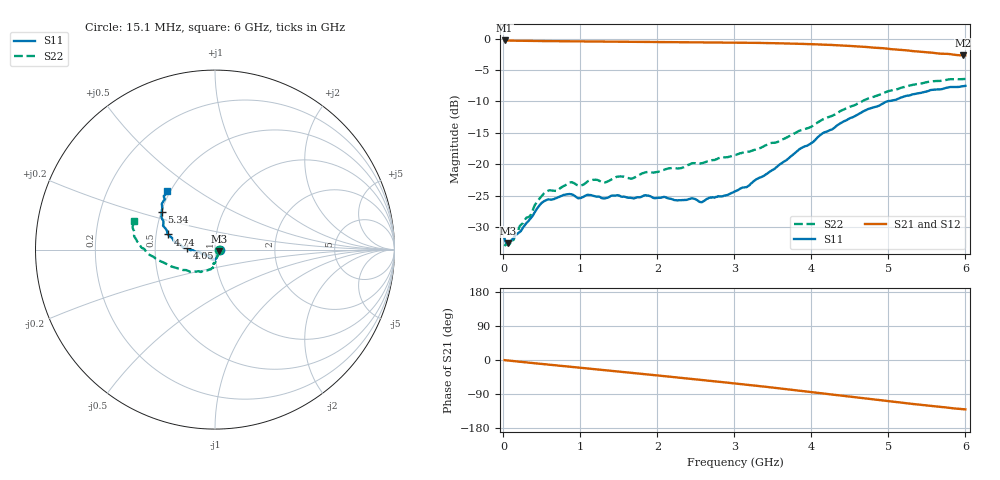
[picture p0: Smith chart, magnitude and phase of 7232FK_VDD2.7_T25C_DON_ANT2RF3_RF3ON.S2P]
!Agilent Technologies,E5071C,MY46417908,A.11.23
!Date: Fri Mar 03 11:30:21 2017
!Data & Calibration Information:
!Freq	S11:SOLT2(ON)	S21:SOLT2(ON)	S12:SOLT2(ON)	S22:SOLT2(ON)
!PortZ  Port1:50+j0  Port2:50+j0
!Above PortZ is port z conversion or system Z0 setting when saving the data.
!When reading, reference impedance value at option line is always used.
# Hz S dB R 50
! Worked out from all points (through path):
!   400 points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, 15.1 MHz to 6 GHz, reference 50 ohm
!   highest |S21| = -0.26 dB at 15.1 MHz (marker M1); lowest = -2.6 dB at 5.97 GHz (marker M2)
!   group delay of S21, straight-line fit = 60.9 ps
!   lowest |S11| = -32.6 dB at 60.1 MHz (marker M3), VSWR 1.05, Z = 52.2 - j0.869 ohm
!   |S11| at or under -10 dB: start of sweep to 4.978 GHz
!   |S22| runs from -33.1 to -6.4 dB; largest |S21 - S12| = 0.0063
!   S11 on the Smith chart (normalised r, x): 15.1 MHz: 1.05, -0.01; 4.05 GHz: 0.73, +0.01; 4.74 GHz: 0.58, +0.11; 5.34 GHz: 0.50, +0.24; 6 GHz: 0.48, +0.38
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1.509975e7  -31.91 -8.7  -0.26 -0.4  -0.25 -0.4  -33.07 -8.8
6.0099e7  -32.61 -20.8  -0.28 -1.4  -0.27 -1.4  -32.90 -23.3
5.40091e8  -25.81 -85.8  -0.36 -11.3  -0.36 -11.3  -24.51 -82.2
6.900885e8  -25.40 -89.1  -0.38 -14.3  -0.38 -14.3  -24.27 -87.7
8.550858e8  -24.75 -95.3  -0.40 -17.6  -0.40 -17.6  -22.92 -90.3
1.020083e9  -25.29 -100.8  -0.41 -20.9  -0.41 -20.9  -23.34 -89.9
1.140081e9  -24.94 -103.5  -0.43 -23.4  -0.43 -23.4  -22.52 -91.0
1.305078e9  -25.47 -107.2  -0.44 -26.7  -0.44 -26.7  -22.94 -91.9
1.485075e9  -24.95 -111.4  -0.46 -30.4  -0.46 -30.4  -21.98 -95.1
1.665072e9  -25.40 -111.4  -0.47 -34.0  -0.47 -34.0  -22.30 -95.1
2.010066e9  -25.37 -117.9  -0.50 -41.0  -0.50 -41.0  -21.21 -94.7
2.460059e9  -25.44 -126.2  -0.54 -50.3  -0.54 -50.3  -19.83 -96.7
2.580057e9  -26.05 -129.8  -0.55 -52.9  -0.55 -52.8  -19.85 -96.5
3.01505e9  -24.30 -149.8  -0.61 -62.1  -0.60 -62.1  -18.53 -107.6
3.165047e9  -23.61 -157.7  -0.64 -65.3  -0.63 -65.3  -18.04 -111.9
4.005033e9  -16.60 178.4  -0.85 -84.7  -0.84 -84.7  -13.97 -145.3
4.050032e9  -16.13 176.7  -0.88 -85.9  -0.87 -85.8  -13.60 -147.0
4.740021e9  -11.18 162.2  -1.33 -102.7  -1.34 -102.6  -9.51 -171.3
5.010016e9  -9.92 155.0  -1.60 -109.0  -1.60 -108.9  -8.31 -178.3
5.340011e9  -8.82 145.0  -1.99 -116.5  -1.98 -116.4  -7.29 174.5
5.97e9  -7.56 129.5  -2.63 -129.6  -2.65 -129.6  -6.43 161.4
6e9  -7.51 129.3  -2.63 -130.3  -2.67 -130.1  -6.40 160.9
